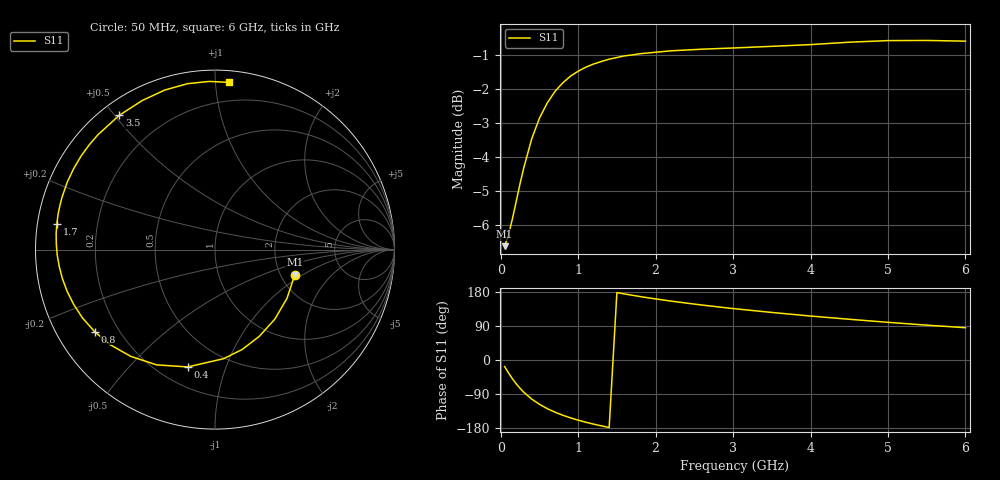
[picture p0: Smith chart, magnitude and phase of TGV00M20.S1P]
! SIEMENS Discrete & RF Semiconductors
! BAT64
! Si Schottky Diode in SOT23
! IF = 0.2 mA
! S-Parameters:  February  1997
# GHz  S  MA  R  50
!  f  S11
! GHz  MAG  ANG
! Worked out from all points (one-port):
!   34 points, 50 MHz to 6 GHz, reference 50 ohm
!   lowest |S11| = -6.6 dB at 50 MHz (marker M1), VSWR 2.75, Z = 119 - j42.5 ohm
!   |S11| at or under -10 dB: nowhere
!   S11 on the Smith chart (normalised r, x): 50 MHz: 2.39, -0.85; 400 MHz: 0.31, -0.75; 800 MHz: 0.11, -0.30; 1.7 GHz: 0.06, +0.08; 3.5 GHz: 0.05, +0.51; 6 GHz: 0.07, +1.08
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0.05  0.4661 -17.4
0.1  0.4843 -34.0
0.15  0.511 -49.2
0.2  0.5427 -63.0
0.25  0.5769 -74.8
0.3  0.6097 -85.5
0.4  0.6712 -103.1
0.5  0.7201 -116.9
0.6  0.7579 -128.3
0.7  0.7883 -137.7
0.8  0.8116 -145.7
0.9  0.8305 -152.6
1  0.8445 -158.8
1.1  0.8563 -164.3
1.3  0.873 -173.8
1.4  0.8797 -178.1
1.6  0.8897 174.2
1.7  0.8925 170.8
2  0.9008 161.2
2.4  0.9076 150.1
2.6  0.9101 145.0
3  0.9137 135.7
3.5  0.919 125.5
4  0.9243 116.0
4.5  0.9319 107.5
5  0.937 99.4
5.5  0.9375 92.0
6  0.9353 85.2
